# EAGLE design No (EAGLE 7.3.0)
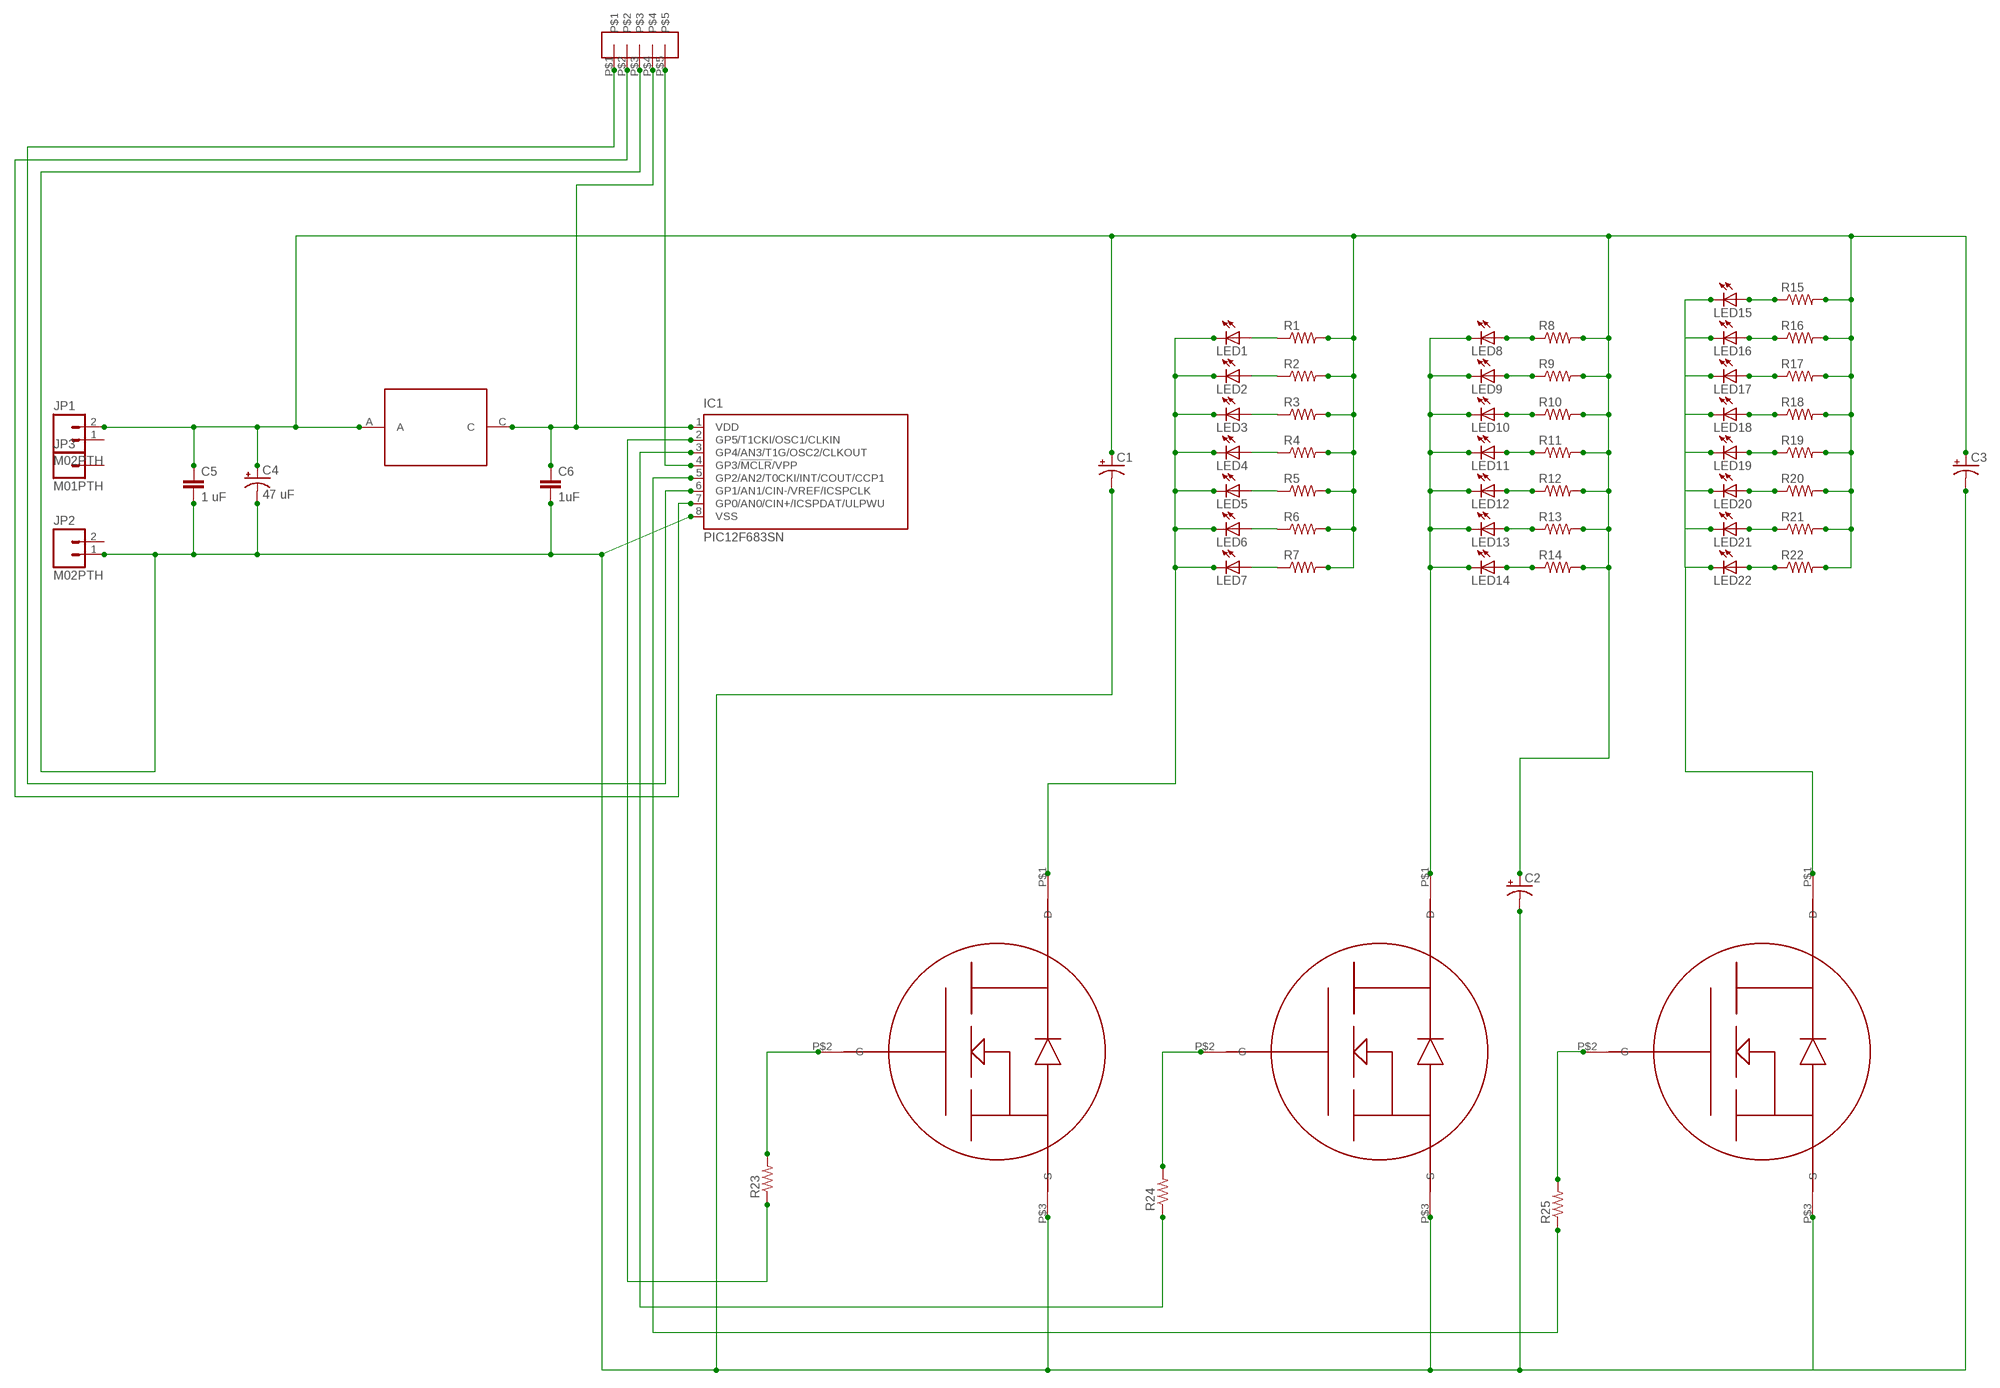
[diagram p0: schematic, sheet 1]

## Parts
C1  CAP_POL3528  [EIA3528]
C2  CAP_POL3528  [EIA3528]
C3  CAP_POL3528  [EIA3528]
C4  47 uF  CAP_POL3528  [EIA3528]
C5  1 uF  CAP1210  [1210]
C6  1uF  CAP1210  [1210]
IC1  PIC12F683SN  [SO-08]
JP1  M02PTH  [1X02]
JP2  M02PTH  [1X02]
JP3  M01PTH  [1X01]
LED1  LED1206  [LED-1206]
LED2  LED1206  [LED-1206]
LED3  LED1206  [LED-1206]
LED4  LED1206  [LED-1206]
LED5  LED1206  [LED-1206]
LED6  LED1206  [LED-1206]
LED7  LED1206  [LED-1206]
LED8  LED1206  [LED-1206]
LED9  LED1206  [LED-1206]
LED10  LED1206  [LED-1206]
LED11  LED1206  [LED-1206]
LED12  LED1206  [LED-1206]
LED13  LED1206  [LED-1206]
LED14  LED1206  [LED-1206]
LED15  LED1206  [LED-1206]
LED16  LED1206  [LED-1206]
LED17  LED1206  [LED-1206]
LED18  LED1206  [LED-1206]
LED19  LED1206  [LED-1206]
LED20  LED1206  [LED-1206]
LED21  LED1206  [LED-1206]
LED22  LED1206  [LED-1206]
R1  RESISTOR0603  [0603-RES]
R2  RESISTOR0603  [0603-RES]
R3  RESISTOR0603  [0603-RES]
R4  RESISTOR0603  [0603-RES]
R5  RESISTOR0603  [0603-RES]
R6  RESISTOR0603  [0603-RES]
R7  RESISTOR0603  [0603-RES]
R8  RESISTOR0603  [0603-RES]
R9  RESISTOR0603  [0603-RES]
R10  RESISTOR0603  [0603-RES]
R11  RESISTOR0603  [0603-RES]
R12  RESISTOR0603  [0603-RES]
R13  RESISTOR0603  [0603-RES]
R14  RESISTOR0603  [0603-RES]
R15  RESISTOR0603  [0603-RES]
R16  RESISTOR0603  [0603-RES]
R17  RESISTOR0603  [0603-RES]
R18  RESISTOR0603  [0603-RES]
R19  RESISTOR0603  [0603-RES]
R20  RESISTOR0603  [0603-RES]
R21  RESISTOR0603  [0603-RES]
R22  RESISTOR0603  [0603-RES]
R23  RESISTOR0603  [0603-RES]
R24  RESISTOR0603  [0603-RES]
R25  RESISTOR0603  [0603-RES]
U$1  IRLML2502  [SOT-23]
U$2  IRLML2502  [SOT-23]
U$3  IRLML2502  [SOT-23]
U$4  ICDP-SMD-2.54  [ICSP-SMD-2-54]
U$5  SM-4007  [SM-4007]

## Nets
N$1: R23.2 U$1.P$2(G)
N$2: IC1.4(GP3/!MCLR!/VPP) U$4.P$5
N$3: LED1.A R1.1
N$4: LED2.A R2.1
N$5: LED3.A R3.1
N$6: LED4.A R4.1
N$7: LED5.A R5.1
N$8: LED6.A R6.1
N$9: LED7.A R7.1
N$10: LED8.A R8.1
N$11: LED9.A R9.1
N$12: LED10.A R10.1
N$13: LED11.A R11.1
N$14: LED12.A R12.1
N$15: LED13.A R13.1
N$16: LED14.A R14.1
N$17: LED22.A R22.1
N$18: LED21.A R21.1
N$19: LED20.A R20.1
N$20: LED19.A R19.1
N$21: LED18.A R18.1
N$22: LED17.A R17.1
N$23: LED16.A R16.1
N$24: LED15.A R15.1
N$25: LED8.C LED9.C LED10.C LED11.C LED12.C LED13.C LED14.C U$2.P$1(D)
N$26: LED15.C LED16.C LED17.C LED18.C LED19.C LED20.C LED21.C LED22.C U$3.P$1(D)
N$27: LED1.C LED2.C LED3.C LED4.C LED5.C LED6.C LED7.C U$1.P$1(D)
N$28: C1.C(-) C2.C(-) C3.C(-) C4.C(-) C5.2 C6.2 IC1.8(VSS) JP2.1 U$1.P$3(S) U$2.P$3(S) U$3.P$3(S) U$4.P$3
N$29: C1.A(+) C2.A(+) C3.A(+) C4.A(+) C5.1 JP1.2 R1.2 R2.2 R3.2 R4.2 R5.2 R6.2 R7.2 R8.2 R9.2 R10.2 R11.2 R12.2 R13.2 R14.2 R15.2 R16.2 R17.2 R18.2 R19.2 R20.2 R21.2 R22.2 U$5.A
N$30: IC1.5(GP2/AN2/T0CKI/INT/COUT/CCP1) R25.1
N$31: IC1.3(GP4/AN3/T1G/OSC2/CLKOUT) R24.1
N$32: IC1.2(GP5/T1CKI/OSC1/CLKIN) R23.1
N$33: R24.2 U$2.P$2(G)
N$34: IC1.7(GP0/AN0/CIN+/ICSPDAT/ULPWU) U$4.P$2
N$35: IC1.6(GP1/AN1/CIN-/VREF/ICSPCLK) U$4.P$1
N$36: R25.2 U$3.P$2(G)
N$38: C6.1 IC1.1(VDD) U$4.P$4 U$5.C
Unconnected: JP1.1 JP2.2 JP3.1

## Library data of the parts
C1-C4 = SparkFun-Capacitors:CAP_POL: Capacitor Polarized
C5 C6 = SparkFun-Capacitors:CAP: Capacitor
IC1 = microchip:PIC12F683: 8-Pin Flash-Based, 8-Bit CMOS Microcontrollers with nanoWatt Technology Source: http://ww1.microchip.com/downloads/en/DeviceDoc/41211D_.pdf; MF: MICROCHIP; MPN: PIC12F683-I/SN; OC_FARNELL: 9759042; OC_NEWARK: 61K3434
JP1 JP2 = SparkFun-Connectors:M02: Standard 2-pin 0.1" header. Use with
JP3 = SparkFun-Connectors:M01: Header 1
LED1-LED22 = SparkFun-LED:LED: LEDs
R1-R25 = SparkFun-Resistors:RESISTOR: Resistor
U$1-U$3 = PonLib:IRLML2502
U$4 = PonLib:ICDP-SMD-2.54
U$5 = PonLib:SM-4007

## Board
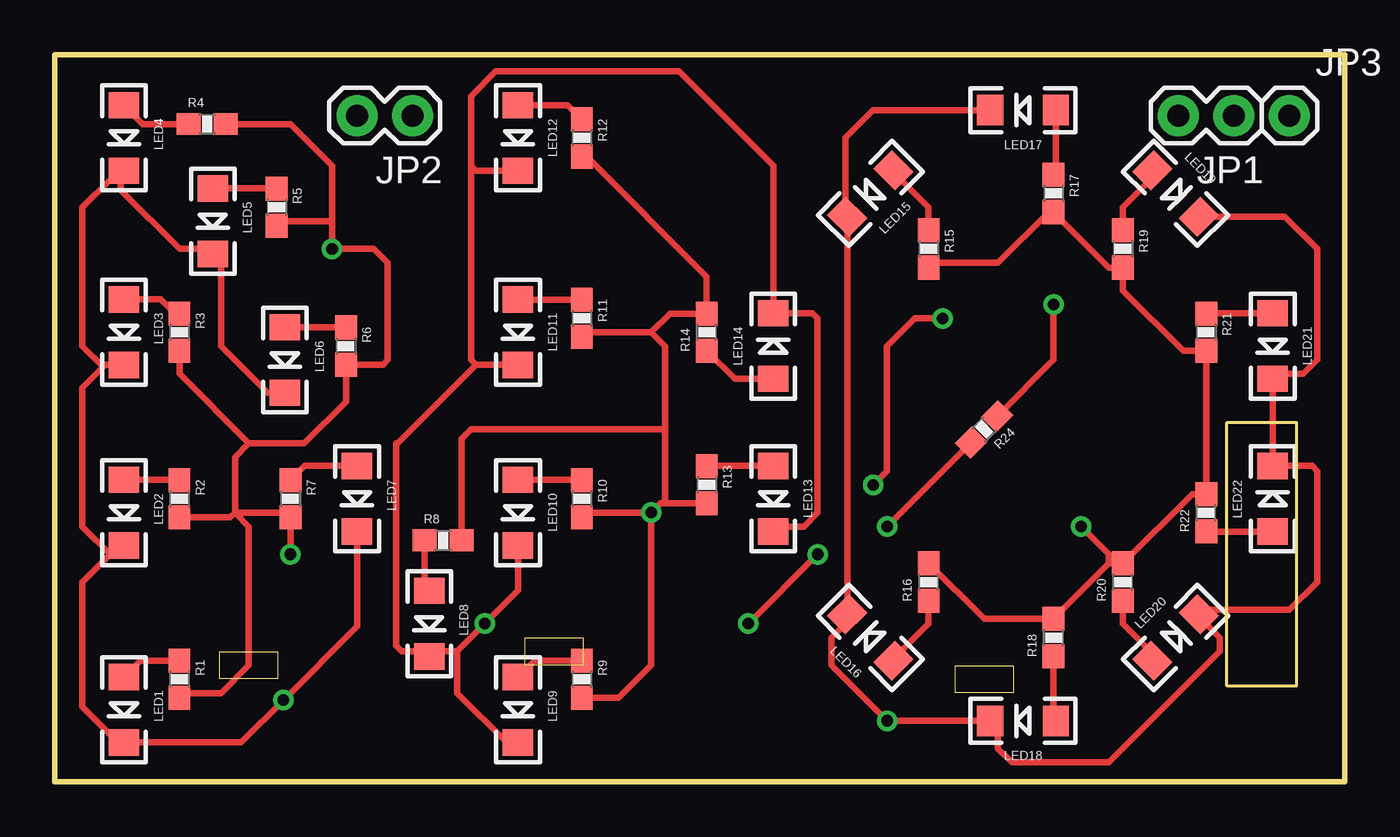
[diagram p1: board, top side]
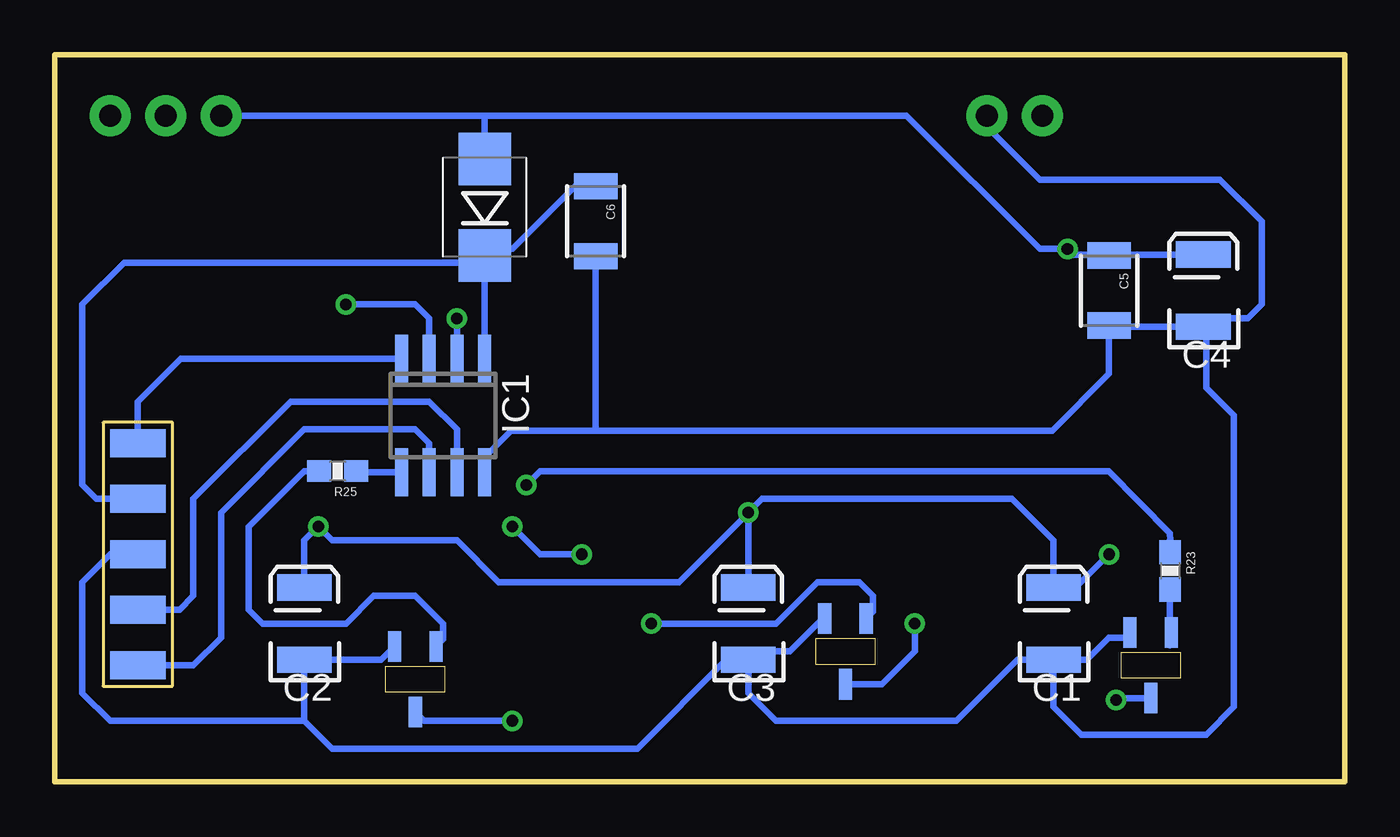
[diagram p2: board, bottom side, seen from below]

Size 59.05 x 33.27 mm. Coordinates in mm from the lower left corner, seen from the top.
Outline: 0,0 59.05,0 59.05,33.27 0,33.27 0,0
Copper layers (1*16): Top 0.035mm / dielectric 1.5mm / Bottom 0.035mm
Design rules "default": minimum track width 10mil, minimum drill 24mil, track to track 8mil, track to pad 8mil, pad to pad 8mil, via to via 8mil, smd to smd 8mil, copper to edge 40mil, drill to drill 8mil, minimum pad ring 10mil, minimum via ring 8mil, stop-mask expansion 4mil, vias tented up to drill 0mil, thermal gap 10mil

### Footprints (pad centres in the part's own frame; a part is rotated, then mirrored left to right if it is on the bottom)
EIA3528 = smd 1.2 x 2.5: A 1.65,0; C -1.65,0
1210 = smd 1.2 x 2: 1 -1.6,0; 2 1.6,0
SO-08 = smd 0.6 x 2.2: 1 -1.905,-2.6; 2 -0.635,-2.6; 3 0.635,-2.6; 4 1.905,-2.6; 5 1.905,2.6; 6 0.635,2.6; 7 -0.635,2.6; 8 -1.905,2.6
1X02 = drill 1.016 pad 1.88: 1 0,0; 2 2.54,0
1X01 = drill 1.016 pad 1.88: 1 0,0
LED-1206 = smd 1.2 x 1.4: A -1.5,0; C 1.5,0
0603-RES = smd 1.1 x 1: 1 -0.85,0; 2 0.85,0
SOT-23 = smd 0.6 x 1.4: P$1 0,1.5; P$2 -0.95,-1.5; P$3 0.95,-1.5
ICSP-SMD-2-54 = smd 2.54 x 1.27: P$1 0,5.08; P$2 0,2.54; P$3 0,0; P$4 0,-2.54; P$5 0,-5.08
SM-4007 = smd 2.4 x 2.4: A 2.2,0; C -2.2,0

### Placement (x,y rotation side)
C1  13.33,7.24 90 bottom
C2  47.62,7.24 90 bottom
C3  27.3,7.24 90 bottom
C4  6.48,22.48 90 bottom
C5  10.79,22.48 270 bottom
C6  34.29,25.65 270 bottom
IC1  41.27,16.76 180 bottom
JP1  53.98,30.48 180 top
JP2  16.38,30.48 180 top
JP3  56.52,30.48 0 top
LED1  3.17,3.3 270 top
LED2  3.17,12.32 270 top
LED3  3.17,20.57 270 top
LED4  3.17,29.46 270 top
LED5  7.24,25.65 270 top
LED6  10.54,19.3 270 top
LED7  13.84,12.95 270 top
LED8  17.15,7.24 270 top
LED9  21.21,3.3 270 top
LED10  21.21,12.32 270 top
LED11  21.21,20.57 270 top
LED12  21.21,29.46 270 top
LED13  32.89,12.95 270 top
LED14  32.89,19.94 90 top
LED15  37.34,26.92 225 top
LED16  37.34,6.6 135 top
LED17  44.32,30.73 180 top
LED18  44.32,2.79 180 top
LED19  51.31,26.92 315 top
LED20  51.31,6.6 45 top
LED21  55.75,19.94 270 top
LED22  55.75,12.95 90 top
R1  5.71,4.7 270 top
R2  5.71,12.95 270 top
R3  5.71,20.57 270 top
R4  6.99,30.1 0 top
R5  10.16,26.29 270 top
R6  13.33,19.94 270 top
R7  10.79,12.95 270 top
R8  17.78,11.05 0 top
R9  24.13,4.7 270 top
R10  24.13,12.95 270 top
R11  24.13,21.21 270 top
R12  24.13,29.46 270 top
R13  29.84,13.59 270 top
R14  29.84,20.57 90 top
R15  40.01,24.38 270 top
R16  40.01,9.14 90 top
R17  45.72,26.92 270 top
R18  45.72,6.6 90 top
R19  48.9,24.38 270 top
R20  48.9,9.14 90 top
R21  52.7,20.57 270 top
R22  52.7,12.32 90 top
R23  8,9.65 270 bottom
R24  42.55,16.13 225 top
R25  46.1,14.22 180 bottom
U$1  8.89,5.33 180 bottom
U$2  22.86,5.97 180 bottom
U$3  42.55,4.7 180 bottom
U$4  55.24,10.41 180 bottom
U$5  39.37,26.29 90 bottom

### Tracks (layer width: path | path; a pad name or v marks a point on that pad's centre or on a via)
N$1
  Bottom 0.305: R23.2 8,6.26 U$1.P$2
N$2
  Bottom 0.305: IC1.4 53.28,19.36 55.24,17.4 U$4.P$5
N$3
  Top 0.305: R1.1 3.92,5.55 LED1.A
N$4
  Top 0.305: LED2.A 5.7,13.82 R2.1
N$5
  Top 0.305: LED3.A 4.85,22.07 5.71,21.21 R3.1
N$6
  Top 0.305: 5.9,30.33 R4.1 4.04,30.1 LED4.A
N$7
  Top 0.305: LED5.A R5.1
N$8
  Top 0.305: LED6.A 13.32,20.8 R6.1
N$9
  Top 0.305: LED7.A 11.44,14.45 R7.1
N$10
  Top 0.305: R8.1 16.93,8.95 LED8.A
N$11
  Top 0.305: R9.1 21.96,5.55 LED9.A
N$12
  Top 0.305: LED10.A 24.12,13.82 R10.1
N$13
  Top 0.305: R11.1 21.22,22.06 LED11.A
N$14
  Top 0.305: 24.12,30.33 R12.1 23.48,30.96 LED12.A
N$15
  Top 0.305: LED13.A 29.86,14.45 R13.1
N$16
  Top 0.305: LED14.A 31.13,18.44 R14.1
N$17
  Top 0.305: LED22.A 52.72,11.45 R22.1
N$18
  Top 0.305: LED21.A 52.72,21.44 R21.1
N$19
  Top 0.305: LED20.A 50.25,5.89 48.9,7.24 R20.1
N$20
  Top 0.305: LED19.A 50.25,27.64 48.9,26.29 R19.1
N$21
  Top 0.305: R18.1 45.72,2.9 LED18.A
N$22
  Top 0.305: LED17.A 45.82,27.88 R17.1
N$23
  Top 0.305: LED16.A 38.4,5.63 40.01,7.24 R16.1
N$24
  Top 0.305: LED15.A 38.4,27.89 40.01,26.29 R15.1
N$25  (via drill 0.53)
  Top 0.305: LED10.C 21.21,8.76 v19.69,7.24 18.41,5.97 | 18.41,5.97 17.38,5.97 LED8.C 16.91,5.97 15.87,5.97 15.62,6.22 15.62,15.49 15.7,15.49 19.28,19.07 | 18.41,5.97 18.41,4.06 20.68,1.8 LED9.C | LED11.C 19.28,19.07 | 19.28,19.07 19.05,19.3 19.05,28.19 | 19.05,28.19 19.05,31.37 20.19,32.51 28.58,32.51 32.89,28.19 LED14.C 34.7,21.44 34.93,21.21 34.93,12.32 34.29,11.68 33.12,11.68 LED13.C | LED12.C 19.28,27.96 19.05,28.19
  Bottom 0.305: U$2.P$1 21.19,4.47 19.69,5.97 v19.69,7.24
N$26  (via drill 0.53)
  Top 0.305: LED17.C 37.47,30.73 36.2,29.46 36.2,25.95 LED15.C LED16.C 36.28,7.32 35.56,6.6 35.56,5.33 v38.1,2.79 LED18.C 43.18,2.44 43.18,1.52 43.82,0.89 48.26,0.89 53.34,5.97 53.34,6.6 52.37,7.57 LED20.C 52.58,7.87 56.52,7.87 57.79,9.14 57.79,14.22 57.55,14.45 LED22.C LED21.C 55.98,18.67 57.15,18.67 57.79,19.3 57.79,24.38 56.31,25.86 LED19.C
  Bottom 0.305: v38.1,2.79 42.14,2.79 U$3.P$1
N$27  (via drill 0.53)
  Top 0.305: LED7.C 13.84,7.11 v10.48,3.75 8.53,1.8 LED1.C 3.15,2.16 2.54,2.16 1.27,3.43 1.27,9.14 2.54,10.41 | LED2.C 2.95,10.82 2.54,10.41 | LED3.C 2.31,19.07 2.22,18.99 | 2.22,18.99 1.27,18.03 1.27,11.68 2.54,10.41 | 2.22,18.99 1.27,19.94 1.27,26.29 2.54,27.56 2.77,27.56 LED4.C 3.02,27.56 3.02,27.07 5.71,24.38 7.01,24.38 LED5.C 7.62,23.77 7.62,19.94 9.76,17.8 LED6.C
  Bottom 0.305: U$1.P$1 10.39,3.83 v10.48,3.75
N$28
  Bottom 0.305: U$2.P$3 23.9,7.47 25.4,5.97 26.93,5.97 C3.C | C3.C 28.32,5.59 32.38,1.52 46.36,1.52 47.62,2.79 | 47.62,2.79 C2.C 44.11,5.59 U$3.P$3 | 13.97,5.59 C1.C 11.81,5.59 10.79,6.6 10.07,6.6 U$1.P$3 | 13.97,5.59 14.99,5.59 17.78,2.79 26.04,2.79 27.3,4.06 C3.C | C4.C 6.1,21.21 4.45,21.21 3.81,21.84 3.81,25.65 5.71,27.56 13.97,27.56 16.38,29.97 JP2.1 | 10.79,20.83 C4.C | C4.C 6.35,20.7 6.35,18.03 5.08,16.76 5.08,3.43 6.35,2.16 12.06,2.16 13.33,3.43 13.33,4.95 13.97,5.59 | C5.2 10.79,18.67 13.4,16.07 34.29,16.07 | U$4.P$3 56.52,10.41 57.79,9.14 57.79,4.06 56.52,2.79 47.62,2.79 | 34.29,16.07 38.16,16.07 39.37,14.86 IC1.8 39.31,14.22 | C6.2 34.29,16.07
  Bottom 0.406: 10.79,20.83 C5.2
N$29  (via drill 0.53)
  Top 0.305: 48.26,9.99 R20.2 52.07,13.17 R22.2 R21.2 51.65,19.72 48.9,22.48 R19.2 48.26,23.53 R17.2 45.51,26.07 43.18,23.75 40.22,23.75 R15.2 | 48.26,9.99 R18.2 42.55,7.45 R16.2 | R12.2 24.34,28.61 29.84,23.11 R14.2 28.16,21.42 27.3,20.57 | 27.3,20.57 24.34,20.57 R11.2 | R13.2 27.94,12.74 | 27.94,12.74 27.73,12.74 v27.3,12.32 | v27.3,12.32 24.34,12.32 R10.2 | 27.94,16.13 27.94,19.94 27.3,20.57 | 27.94,16.13 27.94,12.74 | R9.2 25.82,3.85 27.3,5.33 v27.3,12.32 | R8.2 18.63,15.71 19.05,16.13 27.94,16.13 | 8.89,15.49 11.43,15.49 13.33,17.4 R6.2 15.03,19.09 15.24,19.3 15.24,23.75 14.6,24.38 v12.7,24.38 12.7,25.65 | 8.89,15.49 8.26,14.86 8.26,12.32 | 8.26,12.32 10.58,12.32 R7.2 v10.79,10.41 | R2.2 8.04,12.1 8.26,12.32 | R3.2 5.71,18.67 8.89,15.49 | R1.2 5.93,4.06 7.62,4.06 8.89,5.33 8.89,11.68 8.26,12.32 | R4.2 10.79,30.1 12.7,28.19 12.7,25.65 | 12.7,25.65 10.37,25.65 R5.2 | 48.26,9.99 48.26,10.41 v46.99,11.68
  Bottom 0.305: v27.3,12.32 C3.A | C2.A 47.62,11.05 v46.99,11.68 46.36,11.05 40.64,11.05 38.73,9.14 30.48,9.14 v27.3,12.32 | v10.79,10.41 12.7,8.51 12.96,8.51 C1.A 13.33,11.05 15.24,12.95 26.67,12.95 v27.3,12.32 | C4.A 10.74,24.13 | 10.74,24.13 C5.1 | 10.74,24.13 12.44,24.13 v12.7,24.38 13.97,24.38 20.07,30.48 39.37,30.48 | 39.37,30.48 JP1.2 | U$5.A 39.37,30.48
N$30
  Bottom 0.305: IC1.5 45.45,14.16 R25.1
N$31  (via drill 0.53)
  Top 0.305: v45.72,21.84 45.72,19.3 R24.1
  Bottom 0.305: IC1.3 41.91,21.21 42.55,21.84 v45.72,21.84
N$32  (via drill 0.53)
  Top 0.305: v40.64,21.21 39.37,21.21 38.1,19.94 38.1,14.22 v37.47,13.59
  Bottom 0.305: v40.64,21.21 IC1.2 | v37.47,13.59 36.83,14.22 10.79,14.22 8,11.37 8,11.05 R23.1
N$33  (via drill 0.53)
  Top 0.305: R24.2 v38.1,11.68 | v34.93,10.41 v31.75,7.24
  Bottom 0.305: v38.1,11.68 36.83,10.41 v34.93,10.41 | v31.75,7.24 26.04,7.24 24.13,9.14 22.23,9.14 21.59,8.51 21.59,7.79 U$2.P$2
N$34
  Bottom 0.305: U$4.P$2 53.34,7.87 52.7,8.51 52.7,12.95 48.26,17.4 41.91,17.4 40.64,16.13 IC1.7
N$35
  Bottom 0.305: U$4.P$1 52.7,5.33 51.44,6.6 51.44,12.32 47.62,16.13 42.55,16.13 41.91,15.49 IC1.6
N$36
  Bottom 0.305: R25.2 47.62,14.22 50.16,11.68 50.16,7.87 49.53,7.24 45.72,7.24 44.45,8.51 42.55,8.51 41.27,7.24 41.27,6.52 U$3.P$2
N$38
  Bottom 0.305: U$5.C IC1.1 | U$4.P$4 57.15,12.95 57.79,13.59 57.79,21.84 55.88,23.75 39.71,23.75 U$5.C | C6.1 35.23,27.25 38.1,24.38 39.08,24.38 U$5.C

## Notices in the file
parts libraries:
SparkFun-LED: Licensing: CC v3.0 Share-Alike You are welcome to use this library for commercial purposes.
